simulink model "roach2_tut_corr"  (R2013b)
settings: Solver=VariableStepDiscrete  SolverMode=SingleTasking  StartTime=0.0  StopTime=100  RelTol=1e-3
undefined symbols (not defined in the file): add_latency, addr_width, Bit, bitfield, BitWidth, bram_latency, burst_size, casper_library_scopes, conv_latency, data_width, DelayLen, fan_latency, FFTSize, FFTStage, getfield, increment, led, Location, Lower, mult_latency, mux_latency, n_bits, n_bits_data, n_inputs, n_streams, n_taps, neg_latency, negate_latency, nsamples, pfb_size, pulse_len, reset_period, ROACH, ROACH2, snapshot, sx475t, sync_period, sync_period_bits, Upper, UseCounter, Width
libraries: xbsIndex_r4 x24444, casper_library_misc x73, xbsReplacements_r4 x34, casper_library_delays x14, xps_library x7
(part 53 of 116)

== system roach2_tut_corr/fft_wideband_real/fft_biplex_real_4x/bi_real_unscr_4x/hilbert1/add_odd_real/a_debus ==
  bus_in : Inport
  reinterpret{1..4} (4 alike) : xbsIndex_r4/Reinterpret  force_arith_type=on  arith_type="Signed  (2's comp)"  force_bin_pt=on  bin_pt=17  block_type=reinterpret
  slice1 : xbsIndex_r4/Slice  nbits=18  boolean_output=off  mode=Upper Bit Location + Width  bit1=-54  base1=MSB of Input  bit0=0  base0=LSB of Input  dbl_ovrd=off  block_type=slice
  slice2 : xbsIndex_r4/Slice  nbits=18  boolean_output=off  mode=Upper Bit Location + Width  bit1=-36  base1=MSB of Input  bit0=0  base0=LSB of Input  dbl_ovrd=off  block_type=slice
  slice3 : xbsIndex_r4/Slice  nbits=18  boolean_output=off  mode=Upper Bit Location + Width  bit1=-18  base1=MSB of Input  bit0=0  base0=LSB of Input  dbl_ovrd=off  block_type=slice
  slice4 : xbsIndex_r4/Slice  nbits=18  boolean_output=off  mode=Upper Bit Location + Width  bit1=0  base1=MSB of Input  bit0=0  base0=LSB of Input  dbl_ovrd=off  block_type=slice
  msb_out4 : Outport
  out3 : Outport  Port=2
  out2 : Outport  Port=3
  lsb_out1 : Outport  Port=4
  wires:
  bus_in/1 -> slice4/1, slice3/1, slice2/1, slice1/1
  slice4/1 -> reinterpret4/1
  reinterpret4/1 -> msb_out4/1
  slice3/1 -> reinterpret3/1
  reinterpret3/1 -> out3/1
  slice2/1 -> reinterpret2/1
  reinterpret2/1 -> out2/1
  slice1/1 -> reinterpret1/1
  reinterpret1/1 -> lsb_out1/1

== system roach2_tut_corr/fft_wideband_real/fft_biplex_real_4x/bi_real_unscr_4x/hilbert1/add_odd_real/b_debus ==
  bus_in : Inport
  reinterpret{1..4} (4 alike) : xbsIndex_r4/Reinterpret  force_arith_type=on  arith_type="Signed  (2's comp)"  force_bin_pt=on  bin_pt=17  block_type=reinterpret
  slice1 : xbsIndex_r4/Slice  nbits=18  boolean_output=off  mode=Upper Bit Location + Width  bit1=-54  base1=MSB of Input  bit0=0  base0=LSB of Input  dbl_ovrd=off  block_type=slice
  slice2 : xbsIndex_r4/Slice  nbits=18  boolean_output=off  mode=Upper Bit Location + Width  bit1=-36  base1=MSB of Input  bit0=0  base0=LSB of Input  dbl_ovrd=off  block_type=slice
  slice3 : xbsIndex_r4/Slice  nbits=18  boolean_output=off  mode=Upper Bit Location + Width  bit1=-18  base1=MSB of Input  bit0=0  base0=LSB of Input  dbl_ovrd=off  block_type=slice
  slice4 : xbsIndex_r4/Slice  nbits=18  boolean_output=off  mode=Upper Bit Location + Width  bit1=0  base1=MSB of Input  bit0=0  base0=LSB of Input  dbl_ovrd=off  block_type=slice
  msb_out4 : Outport
  out3 : Outport  Port=2
  out2 : Outport  Port=3
  lsb_out1 : Outport  Port=4
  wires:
  bus_in/1 -> slice4/1, slice3/1, slice2/1, slice1/1
  slice4/1 -> reinterpret4/1
  reinterpret4/1 -> msb_out4/1
  slice3/1 -> reinterpret3/1
  reinterpret3/1 -> out3/1
  slice2/1 -> reinterpret2/1
  reinterpret2/1 -> out2/1
  slice1/1 -> reinterpret1/1
  reinterpret1/1 -> lsb_out1/1

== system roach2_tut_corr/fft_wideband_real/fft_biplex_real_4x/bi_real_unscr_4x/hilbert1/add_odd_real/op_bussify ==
  in1 : Inport
  in2 : Inport  Port=2
  in3 : Inport  Port=3
  in4 : Inport  Port=4
  concatenate : xbsIndex_r4/Concat  num_inputs=4  dbl_ovrd=off  block_type=concat
  reinterpret{1..4} (4 alike) : xbsIndex_r4/Reinterpret  force_arith_type=on  arith_type=Unsigned  force_bin_pt=on  bin_pt=0  block_type=reinterpret
  bus_out : Outport
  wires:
  concatenate/1 -> bus_out/1
  in1/1 -> reinterpret1/1
  reinterpret1/1 -> concatenate/1
  in2/1 -> reinterpret2/1
  reinterpret2/1 -> concatenate/2
  in3/1 -> reinterpret3/1
  reinterpret3/1 -> concatenate/3
  in4/1 -> reinterpret4/1
  reinterpret4/1 -> concatenate/4

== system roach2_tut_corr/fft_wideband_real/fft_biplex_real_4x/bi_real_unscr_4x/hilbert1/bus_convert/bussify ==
  in1 : Inport
  in2 : Inport  Port=2
  in3 : Inport  Port=3
  in4 : Inport  Port=4
  in5 : Inport  Port=5
  in6 : Inport  Port=6
  in7 : Inport  Port=7
  in8 : Inport  Port=8
  in9 : Inport  Port=9
  in10 : Inport  Port=10
  in11 : Inport  Port=11
  in12 : Inport  Port=12
  in13 : Inport  Port=13
  in14 : Inport  Port=14
  in15 : Inport  Port=15
  in16 : Inport  Port=16
  concatenate : xbsIndex_r4/Concat  num_inputs=16  dbl_ovrd=off  block_type=concat
  reinterpret{1..16} (16 alike) : xbsIndex_r4/Reinterpret  force_arith_type=on  arith_type=Unsigned  force_bin_pt=on  bin_pt=0  block_type=reinterpret
  bus_out : Outport
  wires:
  concatenate/1 -> bus_out/1
  in1/1 -> reinterpret1/1
  reinterpret1/1 -> concatenate/1
  in2/1 -> reinterpret2/1
  reinterpret2/1 -> concatenate/2
  in3/1 -> reinterpret3/1
  reinterpret3/1 -> concatenate/3
  in4/1 -> reinterpret4/1
  reinterpret4/1 -> concatenate/4
  in5/1 -> reinterpret5/1
  reinterpret5/1 -> concatenate/5
  in6/1 -> reinterpret6/1
  reinterpret6/1 -> concatenate/6
  in7/1 -> reinterpret7/1
  reinterpret7/1 -> concatenate/7
  in8/1 -> reinterpret8/1
  reinterpret8/1 -> concatenate/8
  in9/1 -> reinterpret9/1
  reinterpret9/1 -> concatenate/9
  in10/1 -> reinterpret10/1
  reinterpret10/1 -> concatenate/10
  in11/1 -> reinterpret11/1
  reinterpret11/1 -> concatenate/11
  in12/1 -> reinterpret12/1
  reinterpret12/1 -> concatenate/12
  in13/1 -> reinterpret13/1
  reinterpret13/1 -> concatenate/13
  in14/1 -> reinterpret14/1
  reinterpret14/1 -> concatenate/14
  in15/1 -> reinterpret15/1
  reinterpret15/1 -> concatenate/15
  in16/1 -> reinterpret16/1
  reinterpret16/1 -> concatenate/16

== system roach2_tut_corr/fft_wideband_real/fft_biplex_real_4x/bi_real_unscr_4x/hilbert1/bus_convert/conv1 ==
  note: (ones_bit & 1) -> round-to-even (ones_bit ^ 1) -> round-to-odd (sign_bit & 1)-> round-to-zero (sign_bit ^ 1) -> round-to-inf (X ~| 1) -> round half down (X | 1) -> round half up
  in : Inport
  Concat : xbsIndex_r4/Concat  num_inputs=2  dbl_ovrd=off  block_type=concat
  Constant : xbsIndex_r4/Constant  const=1  gui_display_data_type=Fixed-point  arith_type=Unsigned  n_bits=1  bin_pt=0  preci_type=Single  exp_width=8  frac_width=24  explicit_period=off  period=1  equ=P=C  opselect=C  inp2=PCIN>>17  opr=+  inp1=P  carry=CIN  dbl_ovrd=off  block_type=constant
  Reinterpret : xbsIndex_r4/Reinterpret  force_arith_type=on  arith_type=Unsigned  force_bin_pt=on  bin_pt=0  block_type=reinterpret
  adder : xbsIndex_r4/AddSub  mode=Addition  use_carryin=off  use_carryout=off  en=off  latency=1  precision=User Defined  arith_type="Signed  (2's comp)"  n_bits=18  bin_pt=17  quantization=Truncate  overflow=Wrap  dbl_ovrd=off  use_behavioral_HDL=off  hw_selection=Fabric  pipelined=on  use_rpm=on  block_type=addsub
  almost_half : xbsIndex_r4/Constant  const=1  gui_display_data_type=Fixed-point  arith_type=Unsigned  n_bits=19  bin_pt=0  preci_type=Single  exp_width=8  frac_width=24  explicit_period=off  period=1  equ=P=C  opselect=C  inp2=PCIN>>17  opr=+  inp1=P  carry=CIN  dbl_ovrd=off  block_type=constant
  bit : xbsIndex_r4/Slice  nbits=1  boolean_output=off  mode=Lower Bit Location + Width  bit1=0  base1=MSB of Input  bit0=1  base0=LSB of Input  dbl_ovrd=off  block_type=slice
  force1 : xbsIndex_r4/Reinterpret  force_arith_type=on  arith_type="Signed  (2's comp)"  force_bin_pt=on  bin_pt=19  block_type=reinterpret
  force2 : xbsIndex_r4/Reinterpret  force_arith_type=off  arith_type="Signed  (2's comp)"  force_bin_pt=on  bin_pt=19  block_type=reinterpret
  tweak_op : xbsIndex_r4/Logical  logical_function=AND  inputs=2  en=off  latency=0  precision=Full  arith_type=Unsigned  n_bits=8  bin_pt=2  align_bp=on  dbl_ovrd=off  block_type=logical
  out : Outport
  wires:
  tweak_op/1 -> Concat/2
  Constant/1 -> tweak_op/2
  bit/1 -> tweak_op/1
  almost_half/1 -> force2/1
  in/1 -> Reinterpret/1, bit/1
  Concat/1 -> force1/1
  Reinterpret/1 -> Concat/1
  force1/1 -> adder/1
  force2/1 -> adder/2
  adder/1 -> out/1

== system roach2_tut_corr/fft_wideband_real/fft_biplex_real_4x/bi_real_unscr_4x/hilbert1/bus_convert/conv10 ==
  note: (ones_bit & 1) -> round-to-even (ones_bit ^ 1) -> round-to-odd (sign_bit & 1)-> round-to-zero (sign_bit ^ 1) -> round-to-inf (X ~| 1) -> round half down (X | 1) -> round half up
  in : Inport
  Concat : xbsIndex_r4/Concat  num_inputs=2  dbl_ovrd=off  block_type=concat
  Constant : xbsIndex_r4/Constant  const=1  gui_display_data_type=Fixed-point  arith_type=Unsigned  n_bits=1  bin_pt=0  preci_type=Single  exp_width=8  frac_width=24  explicit_period=off  period=1  equ=P=C  opselect=C  inp2=PCIN>>17  opr=+  inp1=P  carry=CIN  dbl_ovrd=off  block_type=constant
  Reinterpret : xbsIndex_r4/Reinterpret  force_arith_type=on  arith_type=Unsigned  force_bin_pt=on  bin_pt=0  block_type=reinterpret
  adder : xbsIndex_r4/AddSub  mode=Addition  use_carryin=off  use_carryout=off  en=off  latency=1  precision=User Defined  arith_type="Signed  (2's comp)"  n_bits=18  bin_pt=17  quantization=Truncate  overflow=Wrap  dbl_ovrd=off  use_behavioral_HDL=off  hw_selection=Fabric  pipelined=on  use_rpm=on  block_type=addsub
  almost_half : xbsIndex_r4/Constant  const=1  gui_display_data_type=Fixed-point  arith_type=Unsigned  n_bits=19  bin_pt=0  preci_type=Single  exp_width=8  frac_width=24  explicit_period=off  period=1  equ=P=C  opselect=C  inp2=PCIN>>17  opr=+  inp1=P  carry=CIN  dbl_ovrd=off  block_type=constant
  bit : xbsIndex_r4/Slice  nbits=1  boolean_output=off  mode=Lower Bit Location + Width  bit1=0  base1=MSB of Input  bit0=1  base0=LSB of Input  dbl_ovrd=off  block_type=slice
  force1 : xbsIndex_r4/Reinterpret  force_arith_type=on  arith_type="Signed  (2's comp)"  force_bin_pt=on  bin_pt=19  block_type=reinterpret
  force2 : xbsIndex_r4/Reinterpret  force_arith_type=off  arith_type="Signed  (2's comp)"  force_bin_pt=on  bin_pt=19  block_type=reinterpret
  tweak_op : xbsIndex_r4/Logical  logical_function=AND  inputs=2  en=off  latency=0  precision=Full  arith_type=Unsigned  n_bits=8  bin_pt=2  align_bp=on  dbl_ovrd=off  block_type=logical
  out : Outport
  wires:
  tweak_op/1 -> Concat/2
  Constant/1 -> tweak_op/2
  bit/1 -> tweak_op/1
  almost_half/1 -> force2/1
  in/1 -> Reinterpret/1, bit/1
  Concat/1 -> force1/1
  Reinterpret/1 -> Concat/1
  force1/1 -> adder/1
  force2/1 -> adder/2
  adder/1 -> out/1

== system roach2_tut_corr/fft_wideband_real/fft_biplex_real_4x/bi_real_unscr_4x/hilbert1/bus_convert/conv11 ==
  note: (ones_bit & 1) -> round-to-even (ones_bit ^ 1) -> round-to-odd (sign_bit & 1)-> round-to-zero (sign_bit ^ 1) -> round-to-inf (X ~| 1) -> round half down (X | 1) -> round half up
  in : Inport
  Concat : xbsIndex_r4/Concat  num_inputs=2  dbl_ovrd=off  block_type=concat
  Constant : xbsIndex_r4/Constant  const=1  gui_display_data_type=Fixed-point  arith_type=Unsigned  n_bits=1  bin_pt=0  preci_type=Single  exp_width=8  frac_width=24  explicit_period=off  period=1  equ=P=C  opselect=C  inp2=PCIN>>17  opr=+  inp1=P  carry=CIN  dbl_ovrd=off  block_type=constant
  Reinterpret : xbsIndex_r4/Reinterpret  force_arith_type=on  arith_type=Unsigned  force_bin_pt=on  bin_pt=0  block_type=reinterpret
  adder : xbsIndex_r4/AddSub  mode=Addition  use_carryin=off  use_carryout=off  en=off  latency=1  precision=User Defined  arith_type="Signed  (2's comp)"  n_bits=18  bin_pt=17  quantization=Truncate  overflow=Wrap  dbl_ovrd=off  use_behavioral_HDL=off  hw_selection=Fabric  pipelined=on  use_rpm=on  block_type=addsub
  almost_half : xbsIndex_r4/Constant  const=1  gui_display_data_type=Fixed-point  arith_type=Unsigned  n_bits=19  bin_pt=0  preci_type=Single  exp_width=8  frac_width=24  explicit_period=off  period=1  equ=P=C  opselect=C  inp2=PCIN>>17  opr=+  inp1=P  carry=CIN  dbl_ovrd=off  block_type=constant
  bit : xbsIndex_r4/Slice  nbits=1  boolean_output=off  mode=Lower Bit Location + Width  bit1=0  base1=MSB of Input  bit0=1  base0=LSB of Input  dbl_ovrd=off  block_type=slice
  force1 : xbsIndex_r4/Reinterpret  force_arith_type=on  arith_type="Signed  (2's comp)"  force_bin_pt=on  bin_pt=19  block_type=reinterpret
  force2 : xbsIndex_r4/Reinterpret  force_arith_type=off  arith_type="Signed  (2's comp)"  force_bin_pt=on  bin_pt=19  block_type=reinterpret
  tweak_op : xbsIndex_r4/Logical  logical_function=AND  inputs=2  en=off  latency=0  precision=Full  arith_type=Unsigned  n_bits=8  bin_pt=2  align_bp=on  dbl_ovrd=off  block_type=logical
  out : Outport
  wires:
  tweak_op/1 -> Concat/2
  Constant/1 -> tweak_op/2
  bit/1 -> tweak_op/1
  almost_half/1 -> force2/1
  in/1 -> Reinterpret/1, bit/1
  Concat/1 -> force1/1
  Reinterpret/1 -> Concat/1
  force1/1 -> adder/1
  force2/1 -> adder/2
  adder/1 -> out/1

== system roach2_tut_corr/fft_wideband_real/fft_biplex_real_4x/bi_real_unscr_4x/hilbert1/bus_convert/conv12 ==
  note: (ones_bit & 1) -> round-to-even (ones_bit ^ 1) -> round-to-odd (sign_bit & 1)-> round-to-zero (sign_bit ^ 1) -> round-to-inf (X ~| 1) -> round half down (X | 1) -> round half up
  in : Inport
  Concat : xbsIndex_r4/Concat  num_inputs=2  dbl_ovrd=off  block_type=concat
  Constant : xbsIndex_r4/Constant  const=1  gui_display_data_type=Fixed-point  arith_type=Unsigned  n_bits=1  bin_pt=0  preci_type=Single  exp_width=8  frac_width=24  explicit_period=off  period=1  equ=P=C  opselect=C  inp2=PCIN>>17  opr=+  inp1=P  carry=CIN  dbl_ovrd=off  block_type=constant
  Reinterpret : xbsIndex_r4/Reinterpret  force_arith_type=on  arith_type=Unsigned  force_bin_pt=on  bin_pt=0  block_type=reinterpret
  adder : xbsIndex_r4/AddSub  mode=Addition  use_carryin=off  use_carryout=off  en=off  latency=1  precision=User Defined  arith_type="Signed  (2's comp)"  n_bits=18  bin_pt=17  quantization=Truncate  overflow=Wrap  dbl_ovrd=off  use_behavioral_HDL=off  hw_selection=Fabric  pipelined=on  use_rpm=on  block_type=addsub
  almost_half : xbsIndex_r4/Constant  const=1  gui_display_data_type=Fixed-point  arith_type=Unsigned  n_bits=19  bin_pt=0  preci_type=Single  exp_width=8  frac_width=24  explicit_period=off  period=1  equ=P=C  opselect=C  inp2=PCIN>>17  opr=+  inp1=P  carry=CIN  dbl_ovrd=off  block_type=constant
  bit : xbsIndex_r4/Slice  nbits=1  boolean_output=off  mode=Lower Bit Location + Width  bit1=0  base1=MSB of Input  bit0=1  base0=LSB of Input  dbl_ovrd=off  block_type=slice
  force1 : xbsIndex_r4/Reinterpret  force_arith_type=on  arith_type="Signed  (2's comp)"  force_bin_pt=on  bin_pt=19  block_type=reinterpret
  force2 : xbsIndex_r4/Reinterpret  force_arith_type=off  arith_type="Signed  (2's comp)"  force_bin_pt=on  bin_pt=19  block_type=reinterpret
  tweak_op : xbsIndex_r4/Logical  logical_function=AND  inputs=2  en=off  latency=0  precision=Full  arith_type=Unsigned  n_bits=8  bin_pt=2  align_bp=on  dbl_ovrd=off  block_type=logical
  out : Outport
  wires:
  tweak_op/1 -> Concat/2
  Constant/1 -> tweak_op/2
  bit/1 -> tweak_op/1
  almost_half/1 -> force2/1
  in/1 -> Reinterpret/1, bit/1
  Concat/1 -> force1/1
  Reinterpret/1 -> Concat/1
  force1/1 -> adder/1
  force2/1 -> adder/2
  adder/1 -> out/1

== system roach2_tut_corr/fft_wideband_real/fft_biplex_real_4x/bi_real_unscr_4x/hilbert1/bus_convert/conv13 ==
  note: (ones_bit & 1) -> round-to-even (ones_bit ^ 1) -> round-to-odd (sign_bit & 1)-> round-to-zero (sign_bit ^ 1) -> round-to-inf (X ~| 1) -> round half down (X | 1) -> round half up
  in : Inport
  Concat : xbsIndex_r4/Concat  num_inputs=2  dbl_ovrd=off  block_type=concat
  Constant : xbsIndex_r4/Constant  const=1  gui_display_data_type=Fixed-point  arith_type=Unsigned  n_bits=1  bin_pt=0  preci_type=Single  exp_width=8  frac_width=24  explicit_period=off  period=1  equ=P=C  opselect=C  inp2=PCIN>>17  opr=+  inp1=P  carry=CIN  dbl_ovrd=off  block_type=constant
  Reinterpret : xbsIndex_r4/Reinterpret  force_arith_type=on  arith_type=Unsigned  force_bin_pt=on  bin_pt=0  block_type=reinterpret
  adder : xbsIndex_r4/AddSub  mode=Addition  use_carryin=off  use_carryout=off  en=off  latency=1  precision=User Defined  arith_type="Signed  (2's comp)"  n_bits=18  bin_pt=17  quantization=Truncate  overflow=Wrap  dbl_ovrd=off  use_behavioral_HDL=off  hw_selection=Fabric  pipelined=on  use_rpm=on  block_type=addsub
  almost_half : xbsIndex_r4/Constant  const=1  gui_display_data_type=Fixed-point  arith_type=Unsigned  n_bits=19  bin_pt=0  preci_type=Single  exp_width=8  frac_width=24  explicit_period=off  period=1  equ=P=C  opselect=C  inp2=PCIN>>17  opr=+  inp1=P  carry=CIN  dbl_ovrd=off  block_type=constant
  bit : xbsIndex_r4/Slice  nbits=1  boolean_output=off  mode=Lower Bit Location + Width  bit1=0  base1=MSB of Input  bit0=1  base0=LSB of Input  dbl_ovrd=off  block_type=slice
  force1 : xbsIndex_r4/Reinterpret  force_arith_type=on  arith_type="Signed  (2's comp)"  force_bin_pt=on  bin_pt=19  block_type=reinterpret
  force2 : xbsIndex_r4/Reinterpret  force_arith_type=off  arith_type="Signed  (2's comp)"  force_bin_pt=on  bin_pt=19  block_type=reinterpret
  tweak_op : xbsIndex_r4/Logical  logical_function=AND  inputs=2  en=off  latency=0  precision=Full  arith_type=Unsigned  n_bits=8  bin_pt=2  align_bp=on  dbl_ovrd=off  block_type=logical
  out : Outport
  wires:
  tweak_op/1 -> Concat/2
  Constant/1 -> tweak_op/2
  bit/1 -> tweak_op/1
  almost_half/1 -> force2/1
  in/1 -> Reinterpret/1, bit/1
  Concat/1 -> force1/1
  Reinterpret/1 -> Concat/1
  force1/1 -> adder/1
  force2/1 -> adder/2
  adder/1 -> out/1

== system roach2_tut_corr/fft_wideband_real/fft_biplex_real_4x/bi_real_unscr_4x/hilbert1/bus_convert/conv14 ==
  note: (ones_bit & 1) -> round-to-even (ones_bit ^ 1) -> round-to-odd (sign_bit & 1)-> round-to-zero (sign_bit ^ 1) -> round-to-inf (X ~| 1) -> round half down (X | 1) -> round half up
  in : Inport
  Concat : xbsIndex_r4/Concat  num_inputs=2  dbl_ovrd=off  block_type=concat
  Constant : xbsIndex_r4/Constant  const=1  gui_display_data_type=Fixed-point  arith_type=Unsigned  n_bits=1  bin_pt=0  preci_type=Single  exp_width=8  frac_width=24  explicit_period=off  period=1  equ=P=C  opselect=C  inp2=PCIN>>17  opr=+  inp1=P  carry=CIN  dbl_ovrd=off  block_type=constant
  Reinterpret : xbsIndex_r4/Reinterpret  force_arith_type=on  arith_type=Unsigned  force_bin_pt=on  bin_pt=0  block_type=reinterpret
  adder : xbsIndex_r4/AddSub  mode=Addition  use_carryin=off  use_carryout=off  en=off  latency=1  precision=User Defined  arith_type="Signed  (2's comp)"  n_bits=18  bin_pt=17  quantization=Truncate  overflow=Wrap  dbl_ovrd=off  use_behavioral_HDL=off  hw_selection=Fabric  pipelined=on  use_rpm=on  block_type=addsub
  almost_half : xbsIndex_r4/Constant  const=1  gui_display_data_type=Fixed-point  arith_type=Unsigned  n_bits=19  bin_pt=0  preci_type=Single  exp_width=8  frac_width=24  explicit_period=off  period=1  equ=P=C  opselect=C  inp2=PCIN>>17  opr=+  inp1=P  carry=CIN  dbl_ovrd=off  block_type=constant
  bit : xbsIndex_r4/Slice  nbits=1  boolean_output=off  mode=Lower Bit Location + Width  bit1=0  base1=MSB of Input  bit0=1  base0=LSB of Input  dbl_ovrd=off  block_type=slice
  force1 : xbsIndex_r4/Reinterpret  force_arith_type=on  arith_type="Signed  (2's comp)"  force_bin_pt=on  bin_pt=19  block_type=reinterpret
  force2 : xbsIndex_r4/Reinterpret  force_arith_type=off  arith_type="Signed  (2's comp)"  force_bin_pt=on  bin_pt=19  block_type=reinterpret
  tweak_op : xbsIndex_r4/Logical  logical_function=AND  inputs=2  en=off  latency=0  precision=Full  arith_type=Unsigned  n_bits=8  bin_pt=2  align_bp=on  dbl_ovrd=off  block_type=logical
  out : Outport
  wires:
  tweak_op/1 -> Concat/2
  Constant/1 -> tweak_op/2
  bit/1 -> tweak_op/1
  almost_half/1 -> force2/1
  in/1 -> Reinterpret/1, bit/1
  Concat/1 -> force1/1
  Reinterpret/1 -> Concat/1
  force1/1 -> adder/1
  force2/1 -> adder/2
  adder/1 -> out/1

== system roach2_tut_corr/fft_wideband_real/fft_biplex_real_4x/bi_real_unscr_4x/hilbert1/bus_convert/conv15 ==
  note: (ones_bit & 1) -> round-to-even (ones_bit ^ 1) -> round-to-odd (sign_bit & 1)-> round-to-zero (sign_bit ^ 1) -> round-to-inf (X ~| 1) -> round half down (X | 1) -> round half up
  in : Inport
  Concat : xbsIndex_r4/Concat  num_inputs=2  dbl_ovrd=off  block_type=concat
  Constant : xbsIndex_r4/Constant  const=1  gui_display_data_type=Fixed-point  arith_type=Unsigned  n_bits=1  bin_pt=0  preci_type=Single  exp_width=8  frac_width=24  explicit_period=off  period=1  equ=P=C  opselect=C  inp2=PCIN>>17  opr=+  inp1=P  carry=CIN  dbl_ovrd=off  block_type=constant
  Reinterpret : xbsIndex_r4/Reinterpret  force_arith_type=on  arith_type=Unsigned  force_bin_pt=on  bin_pt=0  block_type=reinterpret
  adder : xbsIndex_r4/AddSub  mode=Addition  use_carryin=off  use_carryout=off  en=off  latency=1  precision=User Defined  arith_type="Signed  (2's comp)"  n_bits=18  bin_pt=17  quantization=Truncate  overflow=Wrap  dbl_ovrd=off  use_behavioral_HDL=off  hw_selection=Fabric  pipelined=on  use_rpm=on  block_type=addsub
  almost_half : xbsIndex_r4/Constant  const=1  gui_display_data_type=Fixed-point  arith_type=Unsigned  n_bits=19  bin_pt=0  preci_type=Single  exp_width=8  frac_width=24  explicit_period=off  period=1  equ=P=C  opselect=C  inp2=PCIN>>17  opr=+  inp1=P  carry=CIN  dbl_ovrd=off  block_type=constant
  bit : xbsIndex_r4/Slice  nbits=1  boolean_output=off  mode=Lower Bit Location + Width  bit1=0  base1=MSB of Input  bit0=1  base0=LSB of Input  dbl_ovrd=off  block_type=slice
  force1 : xbsIndex_r4/Reinterpret  force_arith_type=on  arith_type="Signed  (2's comp)"  force_bin_pt=on  bin_pt=19  block_type=reinterpret
  force2 : xbsIndex_r4/Reinterpret  force_arith_type=off  arith_type="Signed  (2's comp)"  force_bin_pt=on  bin_pt=19  block_type=reinterpret
  tweak_op : xbsIndex_r4/Logical  logical_function=AND  inputs=2  en=off  latency=0  precision=Full  arith_type=Unsigned  n_bits=8  bin_pt=2  align_bp=on  dbl_ovrd=off  block_type=logical
  out : Outport
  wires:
  tweak_op/1 -> Concat/2
  Constant/1 -> tweak_op/2
  bit/1 -> tweak_op/1
  almost_half/1 -> force2/1
  in/1 -> Reinterpret/1, bit/1
  Concat/1 -> force1/1
  Reinterpret/1 -> Concat/1
  force1/1 -> adder/1
  force2/1 -> adder/2
  adder/1 -> out/1

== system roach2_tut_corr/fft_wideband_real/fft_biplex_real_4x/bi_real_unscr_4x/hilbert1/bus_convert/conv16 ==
  note: (ones_bit & 1) -> round-to-even (ones_bit ^ 1) -> round-to-odd (sign_bit & 1)-> round-to-zero (sign_bit ^ 1) -> round-to-inf (X ~| 1) -> round half down (X | 1) -> round half up
  in : Inport
  Concat : xbsIndex_r4/Concat  num_inputs=2  dbl_ovrd=off  block_type=concat
  Constant : xbsIndex_r4/Constant  const=1  gui_display_data_type=Fixed-point  arith_type=Unsigned  n_bits=1  bin_pt=0  preci_type=Single  exp_width=8  frac_width=24  explicit_period=off  period=1  equ=P=C  opselect=C  inp2=PCIN>>17  opr=+  inp1=P  carry=CIN  dbl_ovrd=off  block_type=constant
  Reinterpret : xbsIndex_r4/Reinterpret  force_arith_type=on  arith_type=Unsigned  force_bin_pt=on  bin_pt=0  block_type=reinterpret
  adder : xbsIndex_r4/AddSub  mode=Addition  use_carryin=off  use_carryout=off  en=off  latency=1  precision=User Defined  arith_type="Signed  (2's comp)"  n_bits=18  bin_pt=17  quantization=Truncate  overflow=Wrap  dbl_ovrd=off  use_behavioral_HDL=off  hw_selection=Fabric  pipelined=on  use_rpm=on  block_type=addsub
  almost_half : xbsIndex_r4/Constant  const=1  gui_display_data_type=Fixed-point  arith_type=Unsigned  n_bits=19  bin_pt=0  preci_type=Single  exp_width=8  frac_width=24  explicit_period=off  period=1  equ=P=C  opselect=C  inp2=PCIN>>17  opr=+  inp1=P  carry=CIN  dbl_ovrd=off  block_type=constant
  bit : xbsIndex_r4/Slice  nbits=1  boolean_output=off  mode=Lower Bit Location + Width  bit1=0  base1=MSB of Input  bit0=1  base0=LSB of Input  dbl_ovrd=off  block_type=slice
  force1 : xbsIndex_r4/Reinterpret  force_arith_type=on  arith_type="Signed  (2's comp)"  force_bin_pt=on  bin_pt=19  block_type=reinterpret
  force2 : xbsIndex_r4/Reinterpret  force_arith_type=off  arith_type="Signed  (2's comp)"  force_bin_pt=on  bin_pt=19  block_type=reinterpret
  tweak_op : xbsIndex_r4/Logical  logical_function=AND  inputs=2  en=off  latency=0  precision=Full  arith_type=Unsigned  n_bits=8  bin_pt=2  align_bp=on  dbl_ovrd=off  block_type=logical
  out : Outport
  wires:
  tweak_op/1 -> Concat/2
  Constant/1 -> tweak_op/2
  bit/1 -> tweak_op/1
  almost_half/1 -> force2/1
  in/1 -> Reinterpret/1, bit/1
  Concat/1 -> force1/1
  Reinterpret/1 -> Concat/1
  force1/1 -> adder/1
  force2/1 -> adder/2
  adder/1 -> out/1

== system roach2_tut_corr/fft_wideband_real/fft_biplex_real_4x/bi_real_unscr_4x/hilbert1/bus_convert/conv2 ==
  note: (ones_bit & 1) -> round-to-even (ones_bit ^ 1) -> round-to-odd (sign_bit & 1)-> round-to-zero (sign_bit ^ 1) -> round-to-inf (X ~| 1) -> round half down (X | 1) -> round half up
  in : Inport
  Concat : xbsIndex_r4/Concat  num_inputs=2  dbl_ovrd=off  block_type=concat
  Constant : xbsIndex_r4/Constant  const=1  gui_display_data_type=Fixed-point  arith_type=Unsigned  n_bits=1  bin_pt=0  preci_type=Single  exp_width=8  frac_width=24  explicit_period=off  period=1  equ=P=C  opselect=C  inp2=PCIN>>17  opr=+  inp1=P  carry=CIN  dbl_ovrd=off  block_type=constant
  Reinterpret : xbsIndex_r4/Reinterpret  force_arith_type=on  arith_type=Unsigned  force_bin_pt=on  bin_pt=0  block_type=reinterpret
  adder : xbsIndex_r4/AddSub  mode=Addition  use_carryin=off  use_carryout=off  en=off  latency=1  precision=User Defined  arith_type="Signed  (2's comp)"  n_bits=18  bin_pt=17  quantization=Truncate  overflow=Wrap  dbl_ovrd=off  use_behavioral_HDL=off  hw_selection=Fabric  pipelined=on  use_rpm=on  block_type=addsub
  almost_half : xbsIndex_r4/Constant  const=1  gui_display_data_type=Fixed-point  arith_type=Unsigned  n_bits=19  bin_pt=0  preci_type=Single  exp_width=8  frac_width=24  explicit_period=off  period=1  equ=P=C  opselect=C  inp2=PCIN>>17  opr=+  inp1=P  carry=CIN  dbl_ovrd=off  block_type=constant
  bit : xbsIndex_r4/Slice  nbits=1  boolean_output=off  mode=Lower Bit Location + Width  bit1=0  base1=MSB of Input  bit0=1  base0=LSB of Input  dbl_ovrd=off  block_type=slice
  force1 : xbsIndex_r4/Reinterpret  force_arith_type=on  arith_type="Signed  (2's comp)"  force_bin_pt=on  bin_pt=19  block_type=reinterpret
  force2 : xbsIndex_r4/Reinterpret  force_arith_type=off  arith_type="Signed  (2's comp)"  force_bin_pt=on  bin_pt=19  block_type=reinterpret
  tweak_op : xbsIndex_r4/Logical  logical_function=AND  inputs=2  en=off  latency=0  precision=Full  arith_type=Unsigned  n_bits=8  bin_pt=2  align_bp=on  dbl_ovrd=off  block_type=logical
  out : Outport
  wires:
  tweak_op/1 -> Concat/2
  Constant/1 -> tweak_op/2
  bit/1 -> tweak_op/1
  almost_half/1 -> force2/1
  in/1 -> Reinterpret/1, bit/1
  Concat/1 -> force1/1
  Reinterpret/1 -> Concat/1
  force1/1 -> adder/1
  force2/1 -> adder/2
  adder/1 -> out/1

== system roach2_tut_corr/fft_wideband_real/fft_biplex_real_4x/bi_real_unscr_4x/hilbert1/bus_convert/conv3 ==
  note: (ones_bit & 1) -> round-to-even (ones_bit ^ 1) -> round-to-odd (sign_bit & 1)-> round-to-zero (sign_bit ^ 1) -> round-to-inf (X ~| 1) -> round half down (X | 1) -> round half up
  in : Inport
  Concat : xbsIndex_r4/Concat  num_inputs=2  dbl_ovrd=off  block_type=concat
  Constant : xbsIndex_r4/Constant  const=1  gui_display_data_type=Fixed-point  arith_type=Unsigned  n_bits=1  bin_pt=0  preci_type=Single  exp_width=8  frac_width=24  explicit_period=off  period=1  equ=P=C  opselect=C  inp2=PCIN>>17  opr=+  inp1=P  carry=CIN  dbl_ovrd=off  block_type=constant
  Reinterpret : xbsIndex_r4/Reinterpret  force_arith_type=on  arith_type=Unsigned  force_bin_pt=on  bin_pt=0  block_type=reinterpret
  adder : xbsIndex_r4/AddSub  mode=Addition  use_carryin=off  use_carryout=off  en=off  latency=1  precision=User Defined  arith_type="Signed  (2's comp)"  n_bits=18  bin_pt=17  quantization=Truncate  overflow=Wrap  dbl_ovrd=off  use_behavioral_HDL=off  hw_selection=Fabric  pipelined=on  use_rpm=on  block_type=addsub
  almost_half : xbsIndex_r4/Constant  const=1  gui_display_data_type=Fixed-point  arith_type=Unsigned  n_bits=19  bin_pt=0  preci_type=Single  exp_width=8  frac_width=24  explicit_period=off  period=1  equ=P=C  opselect=C  inp2=PCIN>>17  opr=+  inp1=P  carry=CIN  dbl_ovrd=off  block_type=constant
  bit : xbsIndex_r4/Slice  nbits=1  boolean_output=off  mode=Lower Bit Location + Width  bit1=0  base1=MSB of Input  bit0=1  base0=LSB of Input  dbl_ovrd=off  block_type=slice
  force1 : xbsIndex_r4/Reinterpret  force_arith_type=on  arith_type="Signed  (2's comp)"  force_bin_pt=on  bin_pt=19  block_type=reinterpret
  force2 : xbsIndex_r4/Reinterpret  force_arith_type=off  arith_type="Signed  (2's comp)"  force_bin_pt=on  bin_pt=19  block_type=reinterpret
  tweak_op : xbsIndex_r4/Logical  logical_function=AND  inputs=2  en=off  latency=0  precision=Full  arith_type=Unsigned  n_bits=8  bin_pt=2  align_bp=on  dbl_ovrd=off  block_type=logical
  out : Outport
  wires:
  tweak_op/1 -> Concat/2
  Constant/1 -> tweak_op/2
  bit/1 -> tweak_op/1
  almost_half/1 -> force2/1
  in/1 -> Reinterpret/1, bit/1
  Concat/1 -> force1/1
  Reinterpret/1 -> Concat/1
  force1/1 -> adder/1
  force2/1 -> adder/2
  adder/1 -> out/1

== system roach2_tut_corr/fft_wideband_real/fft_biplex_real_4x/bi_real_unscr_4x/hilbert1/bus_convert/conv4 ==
  note: (ones_bit & 1) -> round-to-even (ones_bit ^ 1) -> round-to-odd (sign_bit & 1)-> round-to-zero (sign_bit ^ 1) -> round-to-inf (X ~| 1) -> round half down (X | 1) -> round half up
  in : Inport
  Concat : xbsIndex_r4/Concat  num_inputs=2  dbl_ovrd=off  block_type=concat
  Constant : xbsIndex_r4/Constant  const=1  gui_display_data_type=Fixed-point  arith_type=Unsigned  n_bits=1  bin_pt=0  preci_type=Single  exp_width=8  frac_width=24  explicit_period=off  period=1  equ=P=C  opselect=C  inp2=PCIN>>17  opr=+  inp1=P  carry=CIN  dbl_ovrd=off  block_type=constant
  Reinterpret : xbsIndex_r4/Reinterpret  force_arith_type=on  arith_type=Unsigned  force_bin_pt=on  bin_pt=0  block_type=reinterpret
  adder : xbsIndex_r4/AddSub  mode=Addition  use_carryin=off  use_carryout=off  en=off  latency=1  precision=User Defined  arith_type="Signed  (2's comp)"  n_bits=18  bin_pt=17  quantization=Truncate  overflow=Wrap  dbl_ovrd=off  use_behavioral_HDL=off  hw_selection=Fabric  pipelined=on  use_rpm=on  block_type=addsub
  almost_half : xbsIndex_r4/Constant  const=1  gui_display_data_type=Fixed-point  arith_type=Unsigned  n_bits=19  bin_pt=0  preci_type=Single  exp_width=8  frac_width=24  explicit_period=off  period=1  equ=P=C  opselect=C  inp2=PCIN>>17  opr=+  inp1=P  carry=CIN  dbl_ovrd=off  block_type=constant
  bit : xbsIndex_r4/Slice  nbits=1  boolean_output=off  mode=Lower Bit Location + Width  bit1=0  base1=MSB of Input  bit0=1  base0=LSB of Input  dbl_ovrd=off  block_type=slice
  force1 : xbsIndex_r4/Reinterpret  force_arith_type=on  arith_type="Signed  (2's comp)"  force_bin_pt=on  bin_pt=19  block_type=reinterpret
  force2 : xbsIndex_r4/Reinterpret  force_arith_type=off  arith_type="Signed  (2's comp)"  force_bin_pt=on  bin_pt=19  block_type=reinterpret
  tweak_op : xbsIndex_r4/Logical  logical_function=AND  inputs=2  en=off  latency=0  precision=Full  arith_type=Unsigned  n_bits=8  bin_pt=2  align_bp=on  dbl_ovrd=off  block_type=logical
  out : Outport
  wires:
  tweak_op/1 -> Concat/2
  Constant/1 -> tweak_op/2
  bit/1 -> tweak_op/1
  almost_half/1 -> force2/1
  in/1 -> Reinterpret/1, bit/1
  Concat/1 -> force1/1
  Reinterpret/1 -> Concat/1
  force1/1 -> adder/1
  force2/1 -> adder/2
  adder/1 -> out/1

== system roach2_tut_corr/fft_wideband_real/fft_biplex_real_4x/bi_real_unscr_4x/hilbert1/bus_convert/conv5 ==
  note: (ones_bit & 1) -> round-to-even (ones_bit ^ 1) -> round-to-odd (sign_bit & 1)-> round-to-zero (sign_bit ^ 1) -> round-to-inf (X ~| 1) -> round half down (X | 1) -> round half up
  in : Inport
  Concat : xbsIndex_r4/Concat  num_inputs=2  dbl_ovrd=off  block_type=concat
  Constant : xbsIndex_r4/Constant  const=1  gui_display_data_type=Fixed-point  arith_type=Unsigned  n_bits=1  bin_pt=0  preci_type=Single  exp_width=8  frac_width=24  explicit_period=off  period=1  equ=P=C  opselect=C  inp2=PCIN>>17  opr=+  inp1=P  carry=CIN  dbl_ovrd=off  block_type=constant
  Reinterpret : xbsIndex_r4/Reinterpret  force_arith_type=on  arith_type=Unsigned  force_bin_pt=on  bin_pt=0  block_type=reinterpret
  adder : xbsIndex_r4/AddSub  mode=Addition  use_carryin=off  use_carryout=off  en=off  latency=1  precision=User Defined  arith_type="Signed  (2's comp)"  n_bits=18  bin_pt=17  quantization=Truncate  overflow=Wrap  dbl_ovrd=off  use_behavioral_HDL=off  hw_selection=Fabric  pipelined=on  use_rpm=on  block_type=addsub
  almost_half : xbsIndex_r4/Constant  const=1  gui_display_data_type=Fixed-point  arith_type=Unsigned  n_bits=19  bin_pt=0  preci_type=Single  exp_width=8  frac_width=24  explicit_period=off  period=1  equ=P=C  opselect=C  inp2=PCIN>>17  opr=+  inp1=P  carry=CIN  dbl_ovrd=off  block_type=constant
  bit : xbsIndex_r4/Slice  nbits=1  boolean_output=off  mode=Lower Bit Location + Width  bit1=0  base1=MSB of Input  bit0=1  base0=LSB of Input  dbl_ovrd=off  block_type=slice
  force1 : xbsIndex_r4/Reinterpret  force_arith_type=on  arith_type="Signed  (2's comp)"  force_bin_pt=on  bin_pt=19  block_type=reinterpret
  force2 : xbsIndex_r4/Reinterpret  force_arith_type=off  arith_type="Signed  (2's comp)"  force_bin_pt=on  bin_pt=19  block_type=reinterpret
  tweak_op : xbsIndex_r4/Logical  logical_function=AND  inputs=2  en=off  latency=0  precision=Full  arith_type=Unsigned  n_bits=8  bin_pt=2  align_bp=on  dbl_ovrd=off  block_type=logical
  out : Outport
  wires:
  tweak_op/1 -> Concat/2
  Constant/1 -> tweak_op/2
  bit/1 -> tweak_op/1
  almost_half/1 -> force2/1
  in/1 -> Reinterpret/1, bit/1
  Concat/1 -> force1/1
  Reinterpret/1 -> Concat/1
  force1/1 -> adder/1
  force2/1 -> adder/2
  adder/1 -> out/1

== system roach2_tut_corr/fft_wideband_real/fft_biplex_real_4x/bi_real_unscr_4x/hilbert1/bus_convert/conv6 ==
  note: (ones_bit & 1) -> round-to-even (ones_bit ^ 1) -> round-to-odd (sign_bit & 1)-> round-to-zero (sign_bit ^ 1) -> round-to-inf (X ~| 1) -> round half down (X | 1) -> round half up
  in : Inport
  Concat : xbsIndex_r4/Concat  num_inputs=2  dbl_ovrd=off  block_type=concat
  Constant : xbsIndex_r4/Constant  const=1  gui_display_data_type=Fixed-point  arith_type=Unsigned  n_bits=1  bin_pt=0  preci_type=Single  exp_width=8  frac_width=24  explicit_period=off  period=1  equ=P=C  opselect=C  inp2=PCIN>>17  opr=+  inp1=P  carry=CIN  dbl_ovrd=off  block_type=constant
  Reinterpret : xbsIndex_r4/Reinterpret  force_arith_type=on  arith_type=Unsigned  force_bin_pt=on  bin_pt=0  block_type=reinterpret
  adder : xbsIndex_r4/AddSub  mode=Addition  use_carryin=off  use_carryout=off  en=off  latency=1  precision=User Defined  arith_type="Signed  (2's comp)"  n_bits=18  bin_pt=17  quantization=Truncate  overflow=Wrap  dbl_ovrd=off  use_behavioral_HDL=off  hw_selection=Fabric  pipelined=on  use_rpm=on  block_type=addsub
  almost_half : xbsIndex_r4/Constant  const=1  gui_display_data_type=Fixed-point  arith_type=Unsigned  n_bits=19  bin_pt=0  preci_type=Single  exp_width=8  frac_width=24  explicit_period=off  period=1  equ=P=C  opselect=C  inp2=PCIN>>17  opr=+  inp1=P  carry=CIN  dbl_ovrd=off  block_type=constant
  bit : xbsIndex_r4/Slice  nbits=1  boolean_output=off  mode=Lower Bit Location + Width  bit1=0  base1=MSB of Input  bit0=1  base0=LSB of Input  dbl_ovrd=off  block_type=slice
  force1 : xbsIndex_r4/Reinterpret  force_arith_type=on  arith_type="Signed  (2's comp)"  force_bin_pt=on  bin_pt=19  block_type=reinterpret
  force2 : xbsIndex_r4/Reinterpret  force_arith_type=off  arith_type="Signed  (2's comp)"  force_bin_pt=on  bin_pt=19  block_type=reinterpret
  tweak_op : xbsIndex_r4/Logical  logical_function=AND  inputs=2  en=off  latency=0  precision=Full  arith_type=Unsigned  n_bits=8  bin_pt=2  align_bp=on  dbl_ovrd=off  block_type=logical
  out : Outport
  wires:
  tweak_op/1 -> Concat/2
  Constant/1 -> tweak_op/2
  bit/1 -> tweak_op/1
  almost_half/1 -> force2/1
  in/1 -> Reinterpret/1, bit/1
  Concat/1 -> force1/1
  Reinterpret/1 -> Concat/1
  force1/1 -> adder/1
  force2/1 -> adder/2
  adder/1 -> out/1

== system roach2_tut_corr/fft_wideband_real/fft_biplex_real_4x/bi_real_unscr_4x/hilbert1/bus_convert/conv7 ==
  note: (ones_bit & 1) -> round-to-even (ones_bit ^ 1) -> round-to-odd (sign_bit & 1)-> round-to-zero (sign_bit ^ 1) -> round-to-inf (X ~| 1) -> round half down (X | 1) -> round half up
  in : Inport
  Concat : xbsIndex_r4/Concat  num_inputs=2  dbl_ovrd=off  block_type=concat
  Constant : xbsIndex_r4/Constant  const=1  gui_display_data_type=Fixed-point  arith_type=Unsigned  n_bits=1  bin_pt=0  preci_type=Single  exp_width=8  frac_width=24  explicit_period=off  period=1  equ=P=C  opselect=C  inp2=PCIN>>17  opr=+  inp1=P  carry=CIN  dbl_ovrd=off  block_type=constant
  Reinterpret : xbsIndex_r4/Reinterpret  force_arith_type=on  arith_type=Unsigned  force_bin_pt=on  bin_pt=0  block_type=reinterpret
  adder : xbsIndex_r4/AddSub  mode=Addition  use_carryin=off  use_carryout=off  en=off  latency=1  precision=User Defined  arith_type="Signed  (2's comp)"  n_bits=18  bin_pt=17  quantization=Truncate  overflow=Wrap  dbl_ovrd=off  use_behavioral_HDL=off  hw_selection=Fabric  pipelined=on  use_rpm=on  block_type=addsub
  almost_half : xbsIndex_r4/Constant  const=1  gui_display_data_type=Fixed-point  arith_type=Unsigned  n_bits=19  bin_pt=0  preci_type=Single  exp_width=8  frac_width=24  explicit_period=off  period=1  equ=P=C  opselect=C  inp2=PCIN>>17  opr=+  inp1=P  carry=CIN  dbl_ovrd=off  block_type=constant
  bit : xbsIndex_r4/Slice  nbits=1  boolean_output=off  mode=Lower Bit Location + Width  bit1=0  base1=MSB of Input  bit0=1  base0=LSB of Input  dbl_ovrd=off  block_type=slice
  force1 : xbsIndex_r4/Reinterpret  force_arith_type=on  arith_type="Signed  (2's comp)"  force_bin_pt=on  bin_pt=19  block_type=reinterpret
  force2 : xbsIndex_r4/Reinterpret  force_arith_type=off  arith_type="Signed  (2's comp)"  force_bin_pt=on  bin_pt=19  block_type=reinterpret
  tweak_op : xbsIndex_r4/Logical  logical_function=AND  inputs=2  en=off  latency=0  precision=Full  arith_type=Unsigned  n_bits=8  bin_pt=2  align_bp=on  dbl_ovrd=off  block_type=logical
  out : Outport
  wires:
  tweak_op/1 -> Concat/2
  Constant/1 -> tweak_op/2
  bit/1 -> tweak_op/1
  almost_half/1 -> force2/1
  in/1 -> Reinterpret/1, bit/1
  Concat/1 -> force1/1
  Reinterpret/1 -> Concat/1
  force1/1 -> adder/1
  force2/1 -> adder/2
  adder/1 -> out/1

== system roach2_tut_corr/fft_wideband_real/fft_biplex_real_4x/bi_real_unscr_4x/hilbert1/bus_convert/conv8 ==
  note: (ones_bit & 1) -> round-to-even (ones_bit ^ 1) -> round-to-odd (sign_bit & 1)-> round-to-zero (sign_bit ^ 1) -> round-to-inf (X ~| 1) -> round half down (X | 1) -> round half up
  in : Inport
  Concat : xbsIndex_r4/Concat  num_inputs=2  dbl_ovrd=off  block_type=concat
  Constant : xbsIndex_r4/Constant  const=1  gui_display_data_type=Fixed-point  arith_type=Unsigned  n_bits=1  bin_pt=0  preci_type=Single  exp_width=8  frac_width=24  explicit_period=off  period=1  equ=P=C  opselect=C  inp2=PCIN>>17  opr=+  inp1=P  carry=CIN  dbl_ovrd=off  block_type=constant
  Reinterpret : xbsIndex_r4/Reinterpret  force_arith_type=on  arith_type=Unsigned  force_bin_pt=on  bin_pt=0  block_type=reinterpret
  adder : xbsIndex_r4/AddSub  mode=Addition  use_carryin=off  use_carryout=off  en=off  latency=1  precision=User Defined  arith_type="Signed  (2's comp)"  n_bits=18  bin_pt=17  quantization=Truncate  overflow=Wrap  dbl_ovrd=off  use_behavioral_HDL=off  hw_selection=Fabric  pipelined=on  use_rpm=on  block_type=addsub
  almost_half : xbsIndex_r4/Constant  const=1  gui_display_data_type=Fixed-point  arith_type=Unsigned  n_bits=19  bin_pt=0  preci_type=Single  exp_width=8  frac_width=24  explicit_period=off  period=1  equ=P=C  opselect=C  inp2=PCIN>>17  opr=+  inp1=P  carry=CIN  dbl_ovrd=off  block_type=constant
  bit : xbsIndex_r4/Slice  nbits=1  boolean_output=off  mode=Lower Bit Location + Width  bit1=0  base1=MSB of Input  bit0=1  base0=LSB of Input  dbl_ovrd=off  block_type=slice
  force1 : xbsIndex_r4/Reinterpret  force_arith_type=on  arith_type="Signed  (2's comp)"  force_bin_pt=on  bin_pt=19  block_type=reinterpret
  force2 : xbsIndex_r4/Reinterpret  force_arith_type=off  arith_type="Signed  (2's comp)"  force_bin_pt=on  bin_pt=19  block_type=reinterpret
  tweak_op : xbsIndex_r4/Logical  logical_function=AND  inputs=2  en=off  latency=0  precision=Full  arith_type=Unsigned  n_bits=8  bin_pt=2  align_bp=on  dbl_ovrd=off  block_type=logical
  out : Outport
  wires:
  tweak_op/1 -> Concat/2
  Constant/1 -> tweak_op/2
  bit/1 -> tweak_op/1
  almost_half/1 -> force2/1
  in/1 -> Reinterpret/1, bit/1
  Concat/1 -> force1/1
  Reinterpret/1 -> Concat/1
  force1/1 -> adder/1
  force2/1 -> adder/2
  adder/1 -> out/1

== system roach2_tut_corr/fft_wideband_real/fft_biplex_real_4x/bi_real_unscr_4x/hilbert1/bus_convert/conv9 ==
  note: (ones_bit & 1) -> round-to-even (ones_bit ^ 1) -> round-to-odd (sign_bit & 1)-> round-to-zero (sign_bit ^ 1) -> round-to-inf (X ~| 1) -> round half down (X | 1) -> round half up
  in : Inport
  Concat : xbsIndex_r4/Concat  num_inputs=2  dbl_ovrd=off  block_type=concat
  Constant : xbsIndex_r4/Constant  const=1  gui_display_data_type=Fixed-point  arith_type=Unsigned  n_bits=1  bin_pt=0  preci_type=Single  exp_width=8  frac_width=24  explicit_period=off  period=1  equ=P=C  opselect=C  inp2=PCIN>>17  opr=+  inp1=P  carry=CIN  dbl_ovrd=off  block_type=constant
  Reinterpret : xbsIndex_r4/Reinterpret  force_arith_type=on  arith_type=Unsigned  force_bin_pt=on  bin_pt=0  block_type=reinterpret
  adder : xbsIndex_r4/AddSub  mode=Addition  use_carryin=off  use_carryout=off  en=off  latency=1  precision=User Defined  arith_type="Signed  (2's comp)"  n_bits=18  bin_pt=17  quantization=Truncate  overflow=Wrap  dbl_ovrd=off  use_behavioral_HDL=off  hw_selection=Fabric  pipelined=on  use_rpm=on  block_type=addsub
  almost_half : xbsIndex_r4/Constant  const=1  gui_display_data_type=Fixed-point  arith_type=Unsigned  n_bits=19  bin_pt=0  preci_type=Single  exp_width=8  frac_width=24  explicit_period=off  period=1  equ=P=C  opselect=C  inp2=PCIN>>17  opr=+  inp1=P  carry=CIN  dbl_ovrd=off  block_type=constant
  bit : xbsIndex_r4/Slice  nbits=1  boolean_output=off  mode=Lower Bit Location + Width  bit1=0  base1=MSB of Input  bit0=1  base0=LSB of Input  dbl_ovrd=off  block_type=slice
  force1 : xbsIndex_r4/Reinterpret  force_arith_type=on  arith_type="Signed  (2's comp)"  force_bin_pt=on  bin_pt=19  block_type=reinterpret
  force2 : xbsIndex_r4/Reinterpret  force_arith_type=off  arith_type="Signed  (2's comp)"  force_bin_pt=on  bin_pt=19  block_type=reinterpret
  tweak_op : xbsIndex_r4/Logical  logical_function=AND  inputs=2  en=off  latency=0  precision=Full  arith_type=Unsigned  n_bits=8  bin_pt=2  align_bp=on  dbl_ovrd=off  block_type=logical
  out : Outport
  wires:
  tweak_op/1 -> Concat/2
  Constant/1 -> tweak_op/2
  bit/1 -> tweak_op/1
  almost_half/1 -> force2/1
  in/1 -> Reinterpret/1, bit/1
  Concat/1 -> force1/1
  Reinterpret/1 -> Concat/1
  force1/1 -> adder/1
  force2/1 -> adder/2
  adder/1 -> out/1

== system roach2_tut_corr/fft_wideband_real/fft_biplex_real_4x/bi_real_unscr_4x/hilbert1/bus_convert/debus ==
  bus_in : Inport
  reinterpret{1..16} (16 alike) : xbsIndex_r4/Reinterpret  force_arith_type=on  arith_type="Signed  (2's comp)"  force_bin_pt=on  bin_pt=18  block_type=reinterpret
  slice1 : xbsIndex_r4/Slice  nbits=19  boolean_output=off  mode=Upper Bit Location + Width  bit1=-285  base1=MSB of Input  bit0=0  base0=LSB of Input  dbl_ovrd=off  block_type=slice
  slice10 : xbsIndex_r4/Slice  nbits=19  boolean_output=off  mode=Upper Bit Location + Width  bit1=-114  base1=MSB of Input  bit0=0  base0=LSB of Input  dbl_ovrd=off  block_type=slice
  slice11 : xbsIndex_r4/Slice  nbits=19  boolean_output=off  mode=Upper Bit Location + Width  bit1=-95  base1=MSB of Input  bit0=0  base0=LSB of Input  dbl_ovrd=off  block_type=slice
  slice12 : xbsIndex_r4/Slice  nbits=19  boolean_output=off  mode=Upper Bit Location + Width  bit1=-76  base1=MSB of Input  bit0=0  base0=LSB of Input  dbl_ovrd=off  block_type=slice
  slice13 : xbsIndex_r4/Slice  nbits=19  boolean_output=off  mode=Upper Bit Location + Width  bit1=-57  base1=MSB of Input  bit0=0  base0=LSB of Input  dbl_ovrd=off  block_type=slice
  slice14 : xbsIndex_r4/Slice  nbits=19  boolean_output=off  mode=Upper Bit Location + Width  bit1=-38  base1=MSB of Input  bit0=0  base0=LSB of Input  dbl_ovrd=off  block_type=slice
  slice15 : xbsIndex_r4/Slice  nbits=19  boolean_output=off  mode=Upper Bit Location + Width  bit1=-19  base1=MSB of Input  bit0=0  base0=LSB of Input  dbl_ovrd=off  block_type=slice
  slice16 : xbsIndex_r4/Slice  nbits=19  boolean_output=off  mode=Upper Bit Location + Width  bit1=0  base1=MSB of Input  bit0=0  base0=LSB of Input  dbl_ovrd=off  block_type=slice
  slice2 : xbsIndex_r4/Slice  nbits=19  boolean_output=off  mode=Upper Bit Location + Width  bit1=-266  base1=MSB of Input  bit0=0  base0=LSB of Input  dbl_ovrd=off  block_type=slice
  slice3 : xbsIndex_r4/Slice  nbits=19  boolean_output=off  mode=Upper Bit Location + Width  bit1=-247  base1=MSB of Input  bit0=0  base0=LSB of Input  dbl_ovrd=off  block_type=slice
  slice4 : xbsIndex_r4/Slice  nbits=19  boolean_output=off  mode=Upper Bit Location + Width  bit1=-228  base1=MSB of Input  bit0=0  base0=LSB of Input  dbl_ovrd=off  block_type=slice
  slice5 : xbsIndex_r4/Slice  nbits=19  boolean_output=off  mode=Upper Bit Location + Width  bit1=-209  base1=MSB of Input  bit0=0  base0=LSB of Input  dbl_ovrd=off  block_type=slice
  slice6 : xbsIndex_r4/Slice  nbits=19  boolean_output=off  mode=Upper Bit Location + Width  bit1=-190  base1=MSB of Input  bit0=0  base0=LSB of Input  dbl_ovrd=off  block_type=slice
  slice7 : xbsIndex_r4/Slice  nbits=19  boolean_output=off  mode=Upper Bit Location + Width  bit1=-171  base1=MSB of Input  bit0=0  base0=LSB of Input  dbl_ovrd=off  block_type=slice
  slice8 : xbsIndex_r4/Slice  nbits=19  boolean_output=off  mode=Upper Bit Location + Width  bit1=-152  base1=MSB of Input  bit0=0  base0=LSB of Input  dbl_ovrd=off  block_type=slice
  slice9 : xbsIndex_r4/Slice  nbits=19  boolean_output=off  mode=Upper Bit Location + Width  bit1=-133  base1=MSB of Input  bit0=0  base0=LSB of Input  dbl_ovrd=off  block_type=slice
  msb_out16 : Outport
  out15 : Outport  Port=2
  out14 : Outport  Port=3
  out13 : Outport  Port=4
  out12 : Outport  Port=5
  out11 : Outport  Port=6
  out10 : Outport  Port=7
  out9 : Outport  Port=8
  out8 : Outport  Port=9
  out7 : Outport  Port=10
  out6 : Outport  Port=11
  out5 : Outport  Port=12
  out4 : Outport  Port=13
  out3 : Outport  Port=14
  out2 : Outport  Port=15
  lsb_out1 : Outport  Port=16
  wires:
  bus_in/1 -> slice16/1, slice15/1, slice14/1, slice13/1, slice12/1, slice11/1, slice10/1, slice9/1, slice8/1, slice7/1, slice6/1, slice5/1, slice4/1, slice3/1, slice2/1, slice1/1
  slice16/1 -> reinterpret16/1
  reinterpret16/1 -> msb_out16/1
  slice15/1 -> reinterpret15/1
  reinterpret15/1 -> out15/1
  slice14/1 -> reinterpret14/1
  reinterpret14/1 -> out14/1
  slice13/1 -> reinterpret13/1
  reinterpret13/1 -> out13/1
  slice12/1 -> reinterpret12/1
  reinterpret12/1 -> out12/1
  slice11/1 -> reinterpret11/1
  reinterpret11/1 -> out11/1
  slice10/1 -> reinterpret10/1
  reinterpret10/1 -> out10/1
  slice9/1 -> reinterpret9/1
  reinterpret9/1 -> out9/1
  slice8/1 -> reinterpret8/1
  reinterpret8/1 -> out8/1
  slice7/1 -> reinterpret7/1
  reinterpret7/1 -> out7/1
  slice6/1 -> reinterpret6/1
  reinterpret6/1 -> out6/1
  slice5/1 -> reinterpret5/1
  reinterpret5/1 -> out5/1
  slice4/1 -> reinterpret4/1
  reinterpret4/1 -> out4/1
  slice3/1 -> reinterpret3/1
  reinterpret3/1 -> out3/1
  slice2/1 -> reinterpret2/1
  reinterpret2/1 -> out2/1
  slice1/1 -> reinterpret1/1
  reinterpret1/1 -> lsb_out1/1
